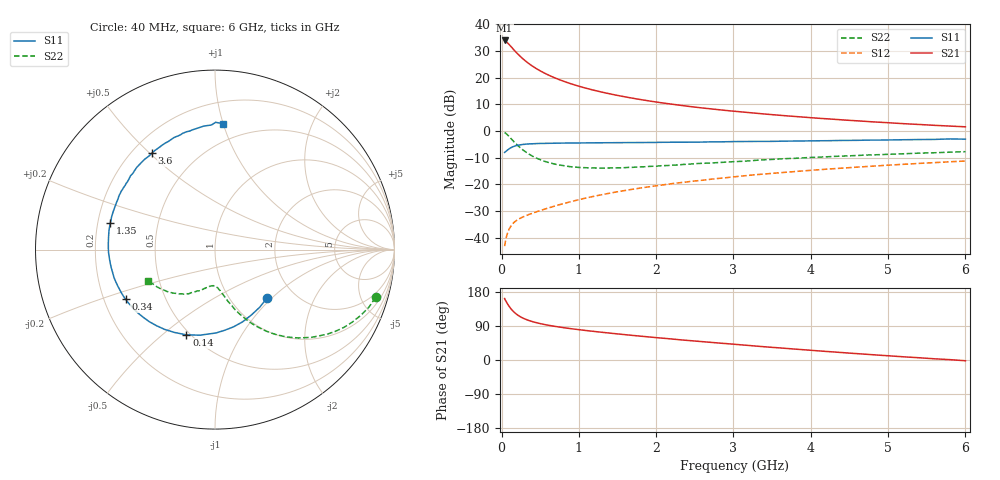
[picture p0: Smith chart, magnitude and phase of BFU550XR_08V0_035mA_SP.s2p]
! Filename:  P:\Prog\Test\Noise\ATS_data\Testdata_Net\03 Spar\BFU550XR_APG2013_45_C05_08p0V_035mA_SP_CM01_D.s2p
! Date/Time: Tue 06/Aug/2013 14:38:18
! BFU550XR_APG2013_45_C05_08p0V_25to35mA_SP_CM01_Bias2_R.s2p
! MDIF S-parameter v. bias file
! BFU550XR_APG2013_45_C05_08p0V_25to35mA_SP_CM01
! Date/time Mon Aug 05 17:22:52 2013
! VAR V_out= 8.0000
! VAR I_out= 35.0000
! VAR V_in= 0.7966
! VAR I_in= 0.3724
! Device data file deembeded for feedlines and parallel
! Original file: \03 Spar\BFU550XR_APG2013_45_C05_08p0V_035mA_SP_CM01_R.s2p
! Feed-files: PR006V01_02082013_Feed1.s2p, PR006V01_02082013_Feed2.s2p
! Parallel-file: PR006V01_02082013_Par.s2p
# MHz S MA R 50
!  Freq-MHz  S11-mag  S11-arg  S21-mag  S21-arg  S12-mag  S12-arg  S22-mag  S22-arg
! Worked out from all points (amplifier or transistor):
!   98 points, 40 MHz to 6 GHz, reference 50 ohm
!   highest |S21| = 34.0 dB at 40 MHz (marker M1)
!   |S21| within 3 dB of that: start of sweep to 144.2 MHz
!   unconditionally stable (mu >= 1): 1.224 GHz to 2.993 GHz
!   at 300 MHz: K = 0.57, MSG = 29.2 dB, |S12| = -32.0 dB
!   at 1.6 GHz: K = 1.02, MAG = 16.6 dB, |S12| = -22.3 dB
!   at 6 GHz: K = 0.86, MSG = 6.4 dB, |S12| = -11.3 dB
!   S11 on the Smith chart (normalised r, x): 40 MHz: 1.46, -0.94; 140 MHz: 0.48, -0.61; 340 MHz: 0.29, -0.24; 1.35 GHz: 0.25, +0.12; 3.6 GHz: 0.28, +0.51; 6 GHz: 0.36, +1.00
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40  0.3962 -43.0  49.85 162.2  0.006914 76.7  0.9331 -16.6
50  0.4066 -52.4  48.51 157.6  0.00843 74.5  0.9156 -20.5
80  0.4427 -76.6  44.59 147.3  0.01243 67.0  0.8387 -31.1
100  0.4643 -89.2  41.55 141.2  0.01456 63.1  0.782 -37.1
120  0.484 -99.9  38.65 135.6  0.01633 59.9  0.7274 -42.2
140  0.501 -108.5  35.87 130.9  0.01786 57.5  0.6766 -46.7
160  0.5138 -116.0  33.2 126.8  0.01915 55.6  0.6312 -50.5
180  0.5257 -122.3  30.88 123.2  0.0203 54.1  0.5887 -53.9
220  0.5433 -132.3  26.95 117.1  0.02216 52.4  0.5179 -59.2
280  0.56 -143.2  22.36 110.3  0.02454 51.6  0.438 -65.1
340  0.5696 -151.0  18.99 105.3  0.02663 51.9  0.3812 -69.3
440  0.5791 -160.2  15.1 99.0  0.03009 53.4  0.3159 -74.0
600  0.5869 -170.1  11.32 91.9  0.03578 56.3  0.2583 -79.4
800  0.5933 -178.4  8.596 85.4  0.0434 59.2  0.2242 -84.1
1050  0.5968 173.6  6.593 78.8  0.05352 61.4  0.2055 -88.5
1350  0.6018 165.9  5.154 72.1  0.06605 62.3  0.2021 -93.5
2050  0.6126 151.2  3.41 58.2  0.09575 61.3  0.2223 -104.0
3100  0.6337 131.6  2.282 40.0  0.1425 56.3  0.2695 -117.7
3600  0.6425 123.3  1.97 31.9  0.1647 52.8  0.299 -124.4
4100  0.6552 114.7  1.733 24.1  0.1873 49.1  0.3229 -130.5
5200  0.6852 97.4  1.371 8.4  0.2372 40.2  0.3739 -144.4
6000  0.7024 86.2  1.197 -2.0  0.2733 33.0  0.4093 -154.9
